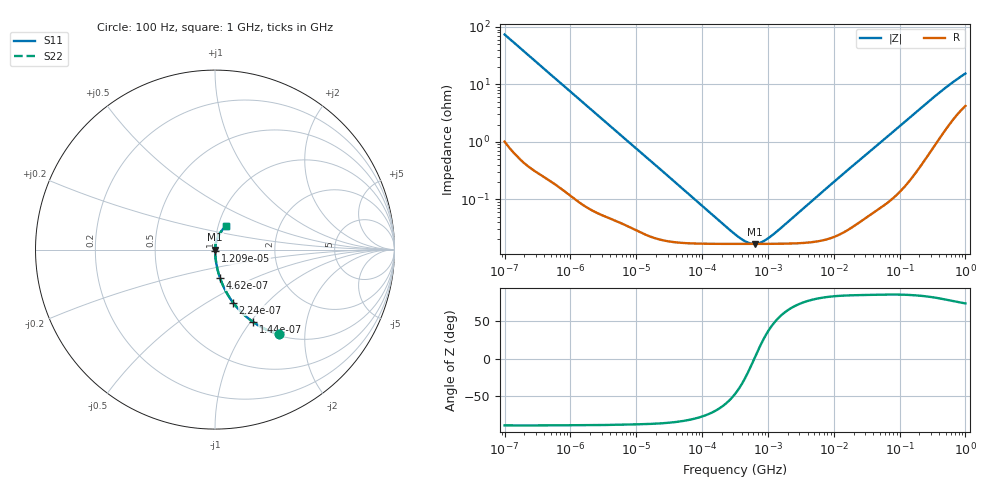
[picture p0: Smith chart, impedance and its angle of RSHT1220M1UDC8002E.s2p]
! RSHT1220M1UDC8002E  S-PARAMETER MODEL  (General Type)
! Model Generated by ELNA Corporation (http://www.ty-top.com)
! Version 1.0
! ELNA Control No.240229
! Copyright (c) 2024 ELNA CO.,LTD. All Rights Reserved.
! Products Name : CONDUCTIVE POLYMER HYBRID ALUMINUM ELECTROLYTIC CAPACITORS
! Characteristics :
!  Capacitance  :  22uF  ,  Rated voltage  :  50V
!  Operating Temp. Range  :  -55 to +105 degC  ,  Endurance  :  10000hr at 105 degC
!  Dimension D  :  6.3mm  ,  Dimension L  :  5.8mm
! Frequency Range : 100Hz - 1GHz
! External Node Assignments :
!  1  o---| |---o  2
# MHz S RI R 50
!Freq[MHz].  S11 Real  S11 Imag  S21 Real  S21 Imag  S12 Real  S12 Imag  S22 Real  S22 Imag
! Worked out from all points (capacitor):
!   401 points, 100 Hz to 1 GHz, reference 50 ohm
!   read as one part in series: C = 21.5 uF near 108 Hz
!   lowest |Z| = 16.8 mohm at 627.3 kHz (marker M1)
!   series resonance near 620.5 kHz, so ESL is about 3.1 nH
!   S11 on the Smith chart (normalised r, x): 100 Hz: 1.02, -1.48; 144 Hz: 1.01, -1.03; 224 Hz: 1.01, -0.66; 462 Hz: 1.00, -0.32; 12.09 kHz: 1.00, -0.01; 1 GHz: 1.08, +0.30
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0.0001  0.3549 -0.4717  0.6451 0.4717  0.6451 0.4717  0.3549 -0.4717
0.000144  0.2119 -0.4028  0.7881 0.4028  0.7881 0.4028  0.2119 -0.4028
0.000183  0.1431 -0.3445  0.8569 0.3445  0.8569 0.3445  0.1431 -0.3445
0.000224  0.1012 -0.2959  0.8988 0.2959  0.8988 0.2959  0.1012 -0.2959
0.000309  0.0568 -0.2254  0.9432 0.2254  0.9432 0.2254  0.0568 -0.2254
0.000462  0.0272 -0.1559  0.9728 0.1559  0.9728 0.1559  0.0272 -0.1559
0.000781  0.0104 -0.0945  0.9896 0.0945  0.9896 0.0945  0.0104 -0.0945
0.001488  0.00335 -0.0502  0.9966 0.0502  0.9966 0.0502  0.00335 -0.0502
0.00361  0.000923 -0.0209  0.9991 0.0209  0.9991 0.0209  0.000923 -0.0209
0.012092  0.0003 -0.00635  0.9997 0.00635  0.9997 0.00635  0.0003 -0.00635
0.022131  0.000213 -0.00348  0.9998 0.00348  0.9998 0.00348  0.000213 -0.00348
0.316228  0.000167 -0.000181  0.9998 0.000181  0.9998 0.000181  0.000167 -0.000181
0.473151  0.000167 -6.85e-05  0.9998 6.85e-05  0.9998 6.85e-05  0.000167 -6.85e-05
0.627336  0.000167 2.77e-06  0.9998 -2.77e-06  0.9998 -2.77e-06  0.000167 2.77e-06
0.798914  0.000168 6.38e-05  0.9998 -6.38e-05  0.9998 -6.38e-05  0.000168 6.38e-05
1.102808  0.000168 0.000152  0.9998 -0.000152  0.9998 -0.000152  0.000168 0.000152
4.704354  0.000181 0.000928  0.9998 -0.000928  0.9998 -0.000928  0.000181 0.000928
69.9842  0.0011 0.0131  0.9989 -0.0131  0.9989 -0.0131  0.0011 0.0131
176.8072  0.00395 0.0324  0.996 -0.0324  0.996 -0.0324  0.00395 0.0324
395.8221  0.0157 0.0681  0.9843 -0.0681  0.9843 -0.0681  0.0157 0.0681
695.825  0.0378 0.1059  0.9622 -0.1059  0.9622 -0.1059  0.0378 0.1059
1000  0.0597 0.1341  0.9403 -0.1341  0.9403 -0.1341  0.0597 0.1341
